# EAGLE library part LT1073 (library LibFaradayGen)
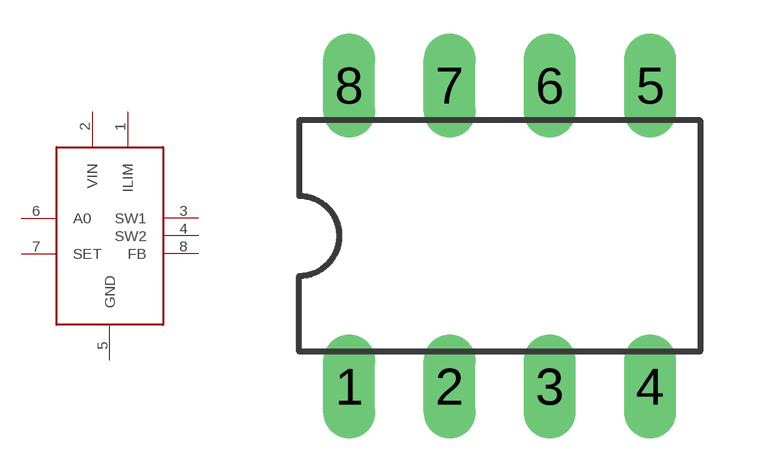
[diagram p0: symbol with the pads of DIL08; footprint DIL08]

Designator prefix -

## LT1073  [DIL08]
1  ILIM
2  VIN
3  SW1
4  SW2
5  GND
6  A0
7  SET
8  FB

## Footprint DIL08 (pad centres in mm)
Dual In Line Package
drill 0.813 long: 1 -3.81,-3.81; 2 -1.27,-3.81; 3 1.27,-3.81; 4 3.81,-3.81; 5 3.81,3.81; 6 1.27,3.81; 7 -1.27,3.81; 8 -3.81,3.81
